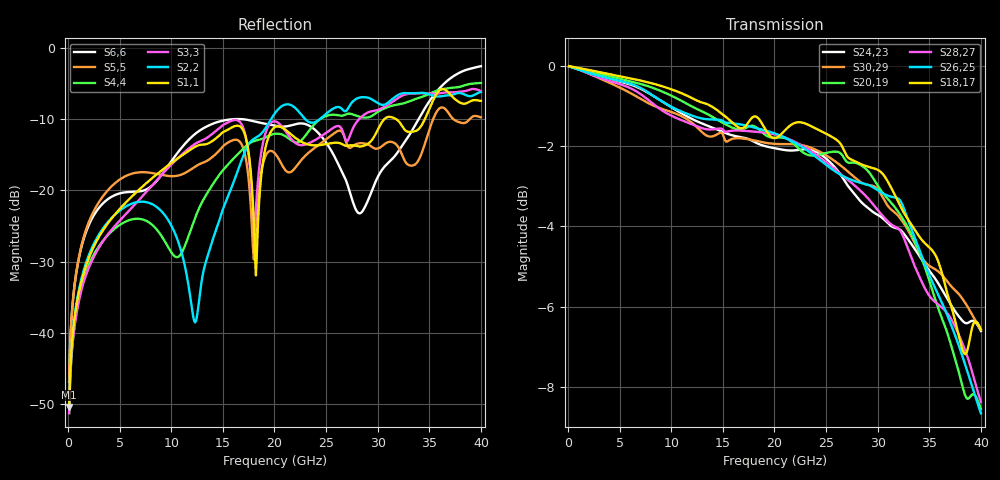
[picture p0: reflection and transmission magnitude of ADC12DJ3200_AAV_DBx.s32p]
! Touchstone file
! Texas Instruments 4/21/2021
! ADC12DJ2700AAV, ADC12DJ3200AAV, ADC08DJ3200AAV
! package type BGA
! High-speed serialized data output for channel B, lane 0-7
# GHZ S MA R 50.000000
! Port[1] = DB0N_BGA_G12
! Port[2] = DB0N_DIE_6
! Port[3] = DB0P_BGA_H12
! Port[4] = DB0P_DIE_5
! Port[5] = DB1N_BGA_J12
! Port[6] = DB1N_DIE_8
! Port[7] = DB1P_BGA_K12
! Port[8] = DB1P_DIE_7
! Port[9] = DB2N_BGA_M11
! Port[10] = DB2N_DIE_10
! Port[11] = DB2P_BGA_M10
! Port[12] = DB2P_DIE_9
! Port[13] = DB3N_BGA_M9
! Port[14] = DB3N_DIE_12
! Port[15] = DB3P_BGA_M8
! Port[16] = DB3P_DIE_11
! Port[17] = DB4N_BGA_G11
! Port[18] = DB4N_DIE_14
! Port[19] = DB4P_BGA_H11
! Port[20] = DB4P_DIE_13
! Port[21] = DB5N_BGA_J11
! Port[22] = DB5N_DIE_16
! Port[23] = DB5P_BGA_K11
! Port[24] = DB5P_DIE_15
! Port[25] = DB6N_BGA_L11
! Port[26] = DB6N_DIE_18
! Port[27] = DB6P_BGA_L10
! Port[28] = DB6P_DIE_17
! Port[29] = DB7N_BGA_L9
! Port[30] = DB7N_DIE_20
! Port[31] = DB7P_BGA_L8
! Port[32] = DB7P_DIE_19
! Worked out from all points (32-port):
!   400 points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, 100 MHz to 40 GHz, reference 50 ohm
!   strongest paths, dB at 100 MHz, 10.1 GHz, 20.1 GHz, 30.1 GHz, 40 GHz:
!     S18,17: 0.0, -0.6, -1.8, -2.6, -6.6
!     S26,25: 0.0, -1.0, -1.7, -3.1, -8.6
!     S28,27: 0.0, -1.3, -1.7, -3.6, -8.4
!     S20,19: 0.0, -0.8, -1.8, -3.0, -8.5
!     S30,29: 0.0, -1.2, -1.9, -3.1, -6.6
!     S24,23: 0.0, -1.0, -2.1, -3.7, -6.6
!   lowest |S11| = -50.3 dB at 100 MHz (marker M1), VSWR 1.01, Z = 50.2 + j0.257 ohm
!   |S11| at or under -10 dB: start of sweep to 30.65 GHz; 31.77 GHz to 34.57 GHz (2.806 GHz wide, 8.46 % of centre)
